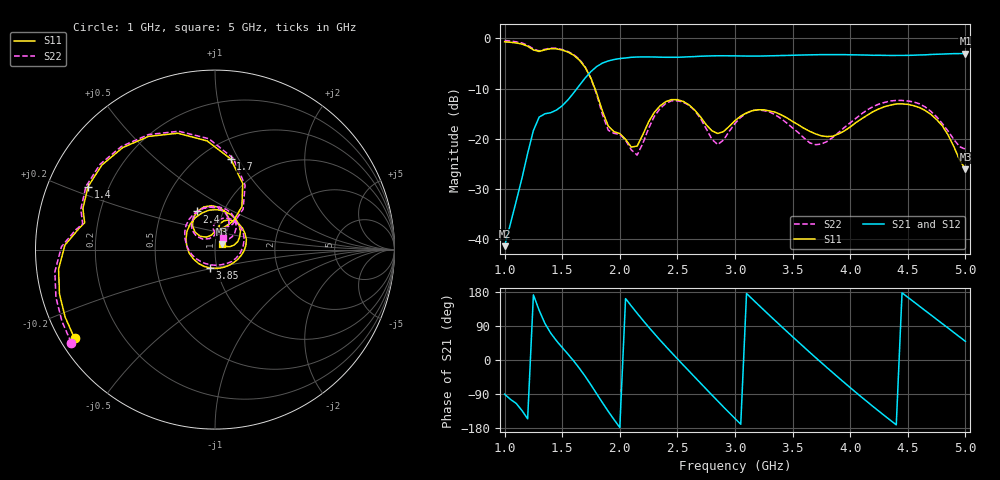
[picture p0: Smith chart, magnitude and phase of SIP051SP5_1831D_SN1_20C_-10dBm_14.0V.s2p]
# GHz  S  dB  R  50
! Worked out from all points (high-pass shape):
!   81 points, 1 GHz to 5 GHz, reference 50 ohm
!   highest |S21| = -3.01 dB at 5 GHz (marker M1); lowest = -41.4 dB at 1 GHz (marker M2)
!   |S21| within 3 dB of the highest: 1.779 GHz to end of sweep
!   lowest |S11| = -26.1 dB at 5 GHz (marker M3), VSWR 1.10, Z = 54.1 + j3.19 ohm
!   |S11| at or under -10 dB: 1.784 GHz to end of sweep
!   |S22| runs from -23.3 to -0.4 dB; largest |S21 - S12| = 0.0022
!   S11 on the Smith chart (normalised r, x): 1 GHz: 0.04, -0.29; 1.4 GHz: 0.12, +0.23; 1.7 GHz: 0.68, +0.93; 2.4 GHz: 0.75, +0.34; 3.85 GHz: 0.92, -0.19; 5 GHz: 1.08, +0.06
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1  -0.67 -147.7  -41.40 -90.2  -41.11 -91.1  -0.41 -147.0
1.25  -2.29 171.4  -18.35 171.9  -18.34 171.8  -2.11 171.9
1.4  -2.05 153.6  -14.80 71.0  -14.81 71.0  -1.93 153.9
1.55  -2.72 120.4  -12.23 15.5  -12.24 15.4  -2.61 120.1
1.7  -5.80 80.2  -7.87 -43.3  -7.89 -43.3  -5.70 78.7
1.85  -14.53 57.3  -4.91 -112.9  -4.91 -113.0  -15.22 55.0
2  -18.96 87.8  -4.02 -178.1  -4.02 -178.1  -19.16 88.2
2.2  -19.16 137.9  -3.69 105.0  -3.69 105.1  -20.93 139.1
2.35  -13.43 124.7  -3.74 52.3  -3.75 52.4  -13.96 130.7
2.4  -12.59 115.1  -3.76 35.7  -3.77 35.5  -12.94 120.1
2.55  -12.55 84.0  -3.72 -13.0  -3.72 -13.0  -12.71 86.1
2.75  -17.20 60.6  -3.51 -76.7  -3.51 -76.7  -17.99 57.7
3  -16.39 78.0  -3.48 -154.4  -3.46 -154.4  -16.94 92.0
3.15  -14.40 57.0  -3.52 161.0  -3.52 161.0  -14.37 66.1
3.35  -14.71 18.1  -3.44 103.5  -3.46 103.5  -15.23 20.0
3.5  -16.54 -13.0  -3.36 61.4  -3.35 61.4  -17.84 -20.4
3.7  -19.03 -59.7  -3.26 6.4  -3.26 6.4  -21.17 -88.3
3.85  -19.49 -106.3  -3.23 -33.7  -3.23 -33.8  -19.70 -140.0
4.1  -16.01 173.6  -3.30 -98.3  -3.30 -98.3  -15.01 160.0
4.35  -13.30 109.8  -3.40 -159.3  -3.40 -159.3  -12.46 111.5
4.7  -15.12 36.1  -3.20 119.1  -3.20 119.2  -14.54 51.6
5  -26.06 36.3  -3.01 49.3  -3.01 49.3  -22.06 56.7
